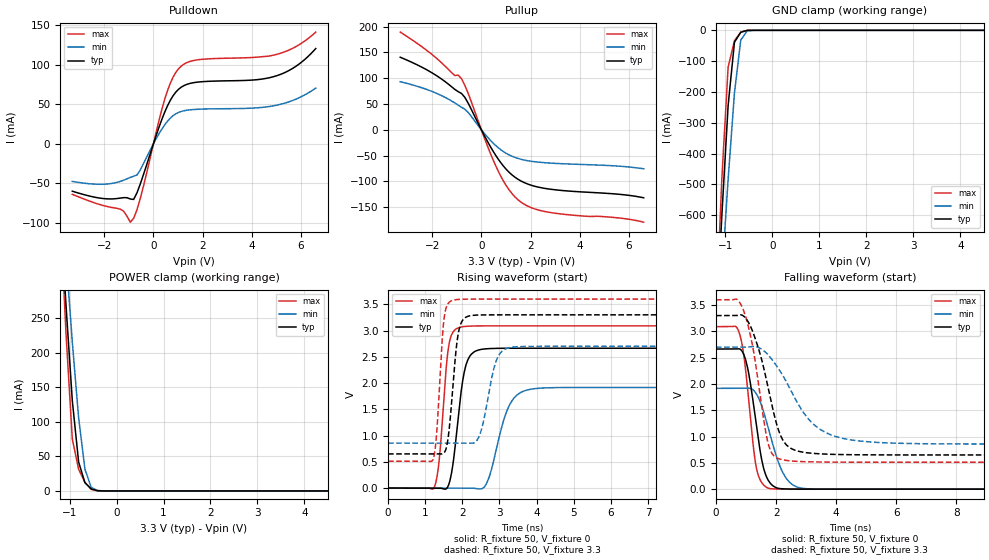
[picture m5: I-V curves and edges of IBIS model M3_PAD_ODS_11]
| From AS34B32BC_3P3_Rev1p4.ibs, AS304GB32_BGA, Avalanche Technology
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[Model] M3_PAD_ODS_11
Model_type I/O
Enable   Active-High
Vinl  =  0.8
Vinh  =  2.2
Vmeas =  1.65
Cref  =  30e-12
| Capacitance  typ   min   max
C_comp   6.058162e-12   5.681079e-12   6.591827e-12
| Variables   typ   min   max
[GND Clamp Reference]   0   0   0
[POWER Clamp Reference]   3.3   2.7   3.6
[Pulldown Reference]   0   0   0
[Pullup Reference]   3.3   2.7   3.6
[Temperature Range]   25   125   -40
[Voltage Range]   3.3   2.7   3.6
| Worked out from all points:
|   slope of the pulldown table from 0 to 0.495 V, typ, clamps not added: 11.6 ohm
|   slope of the pullup table from 0 to 0.495 V, typ, clamps not added: 11.6 ohm
|   GND clamp passes 1 mA (typ) near -0.55 V on its own axis
|   POWER clamp passes 1 mA (typ) near -0.44 V on its own axis
|   falling waveform, R_fixture 50, V_fixture 0: 20-80 % time 420ps typ, 615ps min, 341ps max; typ from 2.66 V to 0 V
|   falling waveform, R_fixture 50, V_fixture 3.3: 20-80 % time 687ps typ, 1.23ns min, 521ps max; typ from 3.3 V to 0.65 V
|   rising waveform, R_fixture 50, V_fixture 0: 20-80 % time 268ps typ, 443ps min, 201ps max; typ from 0 V to 2.66 V
|   rising waveform, R_fixture 50, V_fixture 3.3: 20-80 % time 199ps typ, 315ps min, 156ps max; typ from 0.65 V to 3.3 V
[GND Clamp]
| Voltage   I(typ)   I(min)   I(max)
-3.3V     -7.845A    -6.789A    -9.429A
-1.21V    -1.003A    -1.135A    -970mA
-1.076V   -602.2mA   -800.5mA   -482.6mA
-941.4mV  -243.3mA   -483.1mA   -119mA
-806.9mV  -38.59mA   -202.8mA   -33.75mA
-672.4mV  -6.344mA   -31.46mA   -5.83mA
-537.9mV  -287.2uA   -2.017mA   -75.02uA
-403.4mV  -2.377uA   -74.3uA    -149.1nA
6.6V      0A         0A         0A
[POWER Clamp]
| Voltage   I(typ)   I(min)   I(max)
-3.3V     3.089A     2.693A     3.722A
-1.21V    423.7mA    470.3mA    418.3mA
-1.076V   269.4mA    340.2mA    228.7mA
-941.4mV  130.8mA    215.7mA    75.29mA
-806.9mV  41.91mA    106.1mA    31.39mA
-672.4mV  11.9mA     31.42mA    12.43mA
-537.9mV  2.843mA    4.992mA    2.292mA
-403.4mV  242.8uA    643.4uA    36.75uA
-269mV    569.5nA    24.47uA    93.03nA
6.6V      0A         0A         0A
[Pulldown]
| Voltage   I(typ)   I(min)   I(max)
-3.3V     -60.24mA   -47.82mA   -64.23mA
-1.345V   -68.96mA   -47.76mA   -83.06mA
-941.4mV  -70.11mA   -42.69mA   -99.52mA
-806.9mV  -70.67mA   -41.24mA   -94.66mA
-537.9mV  -51.24mA   -33.31mA   -69.64mA
455.2mV   39.84mA    23.83mA    56.08mA
682.8mV   54.89mA    32.35mA    76.58mA
1.024V    69.09mA    39.7mA     95.16mA
1.821V    78.16mA    43.68mA    106.4mA
4.914V    85.23mA    48.22mA    112.5mA
5.783V    97.9mA     56.32mA    122.9mA
6.6V      120.6mA    70.51mA    141.5mA
[Pullup]
| Voltage   I(typ)   I(min)   I(max)
-3.3V     140.6mA    93.2mA     189.3mA
-1.883V   106.7mA    71.93mA    140.9mA
-1.076V   78.15mA    51.9mA     105.1mA
-941.4mV  73.93mA    47.76mA    105.9mA
-806.9mV  70.38mA    43.76mA    98.84mA
-537.9mV  51.76mA    33.91mA    70.85mA
227.6mV   -20.67mA   -12.99mA   -28.83mA
682.8mV   -56.54mA   -34.48mA   -79.66mA
1.138V    -82.63mA   -48.76mA   -116.9mA
1.593V    -98.59mA   -56.76mA   -139.3mA
2.731V    -114.5mA   -64.15mA   -159.5mA
6.6V      -131.6mA   -75.43mA   -178.8mA
[Ramp]
dV/dt_r   1.59832/0.268001n  1.14988/0.442819n  1.85402/0.201498n
dV/dt_f   1.58992/0.687394n  1.10595/1.2346n  1.85299/0.520805n
R_load = 50
[Falling Waveform]
R_fixture = 50
V_fixture = 0
V_fixture_min = 0
V_fixture_max = 0
| Time   V(typ)   V(min)   V(max)
0s        2.664V     1.916V     3.09V
685ps     2.666V     1.917V     3.079V
948.1ps   2.528V     1.917V     2.451V
1.113ns   2.124V     1.919V     1.549V
1.359ns   1.15V      1.8V       364.3mV
1.565ns   446mV      1.512V     93.74mV
1.816ns   107.7mV    1.004V     8.676mV
2.285ns   4.678mV    253mV      1.259mV
2.925ns   778.8uV    12.55mV    466uV
21.88ns   1.332uV    701.6nV    -2.001uV
[Falling Waveform]
R_fixture = 50
V_fixture = 3.3
V_fixture_min = 2.7
V_fixture_max = 3.6
| Time   V(typ)   V(min)   V(max)
0s        3.3V       2.7V       3.6V
684.8ps   3.301V     2.7V       3.611V
919.3ps   3.291V     2.701V     3.395V
1.226ns   2.993V     2.712V     2.699V
1.721ns   1.965V     2.562V     905.3mV
2.171ns   993.9mV    2.21V      564.8mV
2.504ns   771.7mV    1.866V     536.3mV
3.285ns   678mV      1.216V     517.6mV
4.744ns   653.6mV    916.9mV    512.4mV
21.88ns   650.1mV    856.8mV    511.7mV
[Rising Waveform]
R_fixture = 50
V_fixture = 0
V_fixture_min = 0
V_fixture_max = 0
| Time   V(typ)   V(min)   V(max)
0s        15.73nV    147.4nV    21.47nV
1.245ns   -582.5uV   -252uV     15.83mV
1.377ns   -644.2uV   -278.7uV   529.1mV
1.636ns   68.32mV    -331.1uV   2.716V
1.945ns   1.706V     -393.8uV   3.064V
2.295ns   2.583V     -2.335mV   3.087V
2.688ns   2.655V     143.9mV    3.09V
3.3ns     2.663V     1.62V      3.09V
3.877ns   2.663V     1.887V     3.09V
21.88ns   2.664V     1.916V     3.09V
[Rising Waveform]
R_fixture = 50
V_fixture = 3.3
V_fixture_min = 2.7
V_fixture_max = 3.6
| Time   V(typ)   V(min)   V(max)
0s        650.1mV    856.8mV    511.7mV
1.212ns   649.7mV    856.3mV    545.4mV
1.304ns   649.6mV    856.2mV    1.001V
1.518ns   679.7mV    856.1mV    3.276V
1.796ns   2.362V     856mV      3.586V
2.057ns   3.235V     855.9mV    3.598V
2.435ns   3.296V     958.8mV    3.599V
2.912ns   3.299V     2.422V     3.599V
3.375ns   3.299V     2.686V     3.599V
21.88ns   3.3V       2.7V       3.6V
